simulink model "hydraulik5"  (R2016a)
settings: Solver=ode45  StartTime=0.0  StopTime=2  MaxStep=0.01  RelTol=1e-3  AbsTol=1e-3
InitFcn:
  | pa = 1e5;
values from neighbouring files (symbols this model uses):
  A = zeros(1,N)    [sfun_inferenz.m]
  alpha = 2e-6    (= 2e-06)    [init_epidemie.m]
  m = 1.0    (= 1)    [init_pendelStange.m]
undefined symbols (not defined in the file or in its folder): Amin, K, p0, Qzu, R, rho, ta, te, V0
libraries: simulink x1

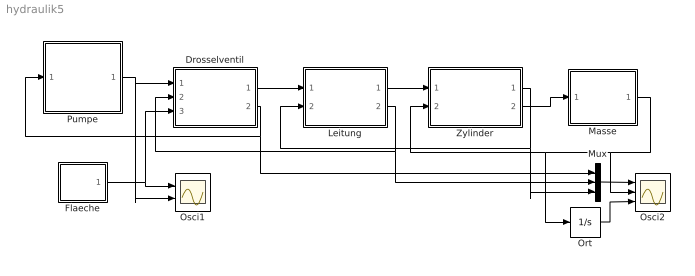
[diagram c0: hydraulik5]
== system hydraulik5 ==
  Drosselventil : Subsystem
  Flaeche : Subsystem
  Leitung : Subsystem
  Masse : Subsystem
  Mux : Mux  Inputs=3
  Ort : Integrator
  Osci1 : Scope  NumInputPorts=2
  Osci2 : Scope  NumInputPorts=3
  Pumpe : Subsystem
  Zylinder : Subsystem
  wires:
  Leitung/2(p1) -> Drosselventil/2(p2), Mux/2
  Leitung/1(Q2) -> Zylinder/1(Q)
  Zylinder/1(p) -> Mux/3, Leitung/2(p2)
  Zylinder/2(F) -> Masse/1(F)
  Masse/1(v) -> Ort/1, Zylinder/2(v), Osci2/2
  Pumpe/1(Q) -> Drosselventil/1(Q1), Osci1/2
  Drosselventil/1(Q2) -> Leitung/1(Q1)
  Drosselventil/2(p1) -> Mux/1, Pumpe/1(p)
  Flaeche/1(Out1) -> Drosselventil/3(A), Osci1/1
  Mux/1 -> Osci2/1
  Ort/1 -> Osci2/3

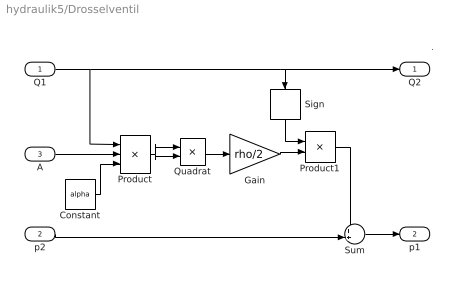
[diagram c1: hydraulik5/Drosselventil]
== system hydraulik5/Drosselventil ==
  note: .
  Q1 : Inport
  p2 : Inport  Port=2
  A : Inport  Port=3
  Constant : Constant  Value=alpha
  Gain : Gain  Gain=rho/2
  Product : Product  Inputs=*//
  Product1 : Product
  Quadrat : Product
  Sign : Signum
  Sum : Sum  Inputs=++|
  Q2 : Outport
  p1 : Outport  Port=2
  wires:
  Sum/1 -> p1/1
  p2/1 -> Sum/2
  Q1/1 -> Product/1, Q2/1, Sign/1
  A/1 -> Product/2
  Constant/1 -> Product/3
  Quadrat/1 -> Gain/1
  Gain/1 -> Product1/2
  Product1/1 -> Sum/1
  Sign/1 -> Product1/1
  Product/1 -> Quadrat/1, Quadrat/2

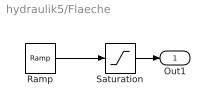
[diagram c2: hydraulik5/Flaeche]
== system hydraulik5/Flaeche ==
  Ramp : simulink/Sources/Ramp  slope=(A-Amin)/(te-ta)  start=ta  X0=0
  Saturation : Saturate  UpperLimit=A  LowerLimit=Amin
  Out1 : Outport
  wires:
  Ramp/1 -> Saturation/1
  Saturation/1 -> Out1/1

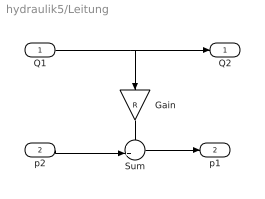
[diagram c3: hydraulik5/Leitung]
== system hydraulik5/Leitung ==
  Q1 : Inport
  p2 : Inport  Port=2
  Gain : Gain  Gain=R
  Sum : Sum  Inputs=++|
  Q2 : Outport
  p1 : Outport  Port=2
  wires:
  Q1/1 -> Q2/1, Gain/1
  p2/1 -> Sum/2
  Sum/1 -> p1/1
  Gain/1 -> Sum/1

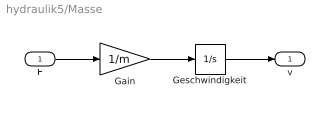
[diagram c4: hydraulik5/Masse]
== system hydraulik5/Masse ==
  F : Inport
  Gain : Gain  Gain=1/m
  Geschwindigkeit : Integrator
  v : Outport
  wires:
  F/1 -> Gain/1
  Geschwindigkeit/1 -> v/1
  Gain/1 -> Geschwindigkeit/1

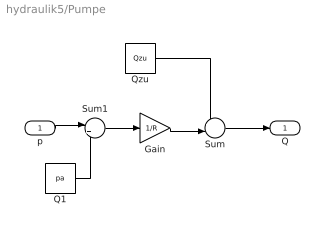
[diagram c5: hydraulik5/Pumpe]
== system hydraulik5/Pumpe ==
  p : Inport
  Gain : Gain  Gain=1/R
  Q1 : Constant  Value=pa
  Qzu : Constant  Value=Qzu
  Sum : Sum  Inputs=+-|
  Sum1 : Sum  Inputs=|+-
  Q : Outport
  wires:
  Qzu/1 -> Sum/1
  Gain/1 -> Sum/2
  Sum/1 -> Q/1
  p/1 -> Sum1/1
  Sum1/1 -> Gain/1
  Q1/1 -> Sum1/2

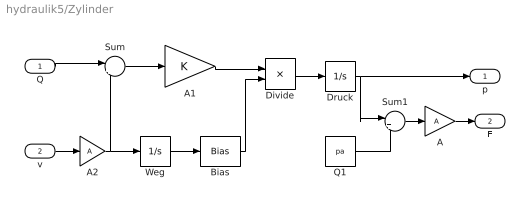
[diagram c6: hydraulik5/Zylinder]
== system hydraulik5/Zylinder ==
  Q : Inport
  v : Inport  Port=2
  A : Gain  Gain=A
  A1 : Gain  Gain=K
  A2 : Gain  Gain=A
  Bias : Bias  Bias=V0
  Divide : Product  Inputs=*/
  Druck : Integrator  InitialCondition=p0  LimitOutput=on  LowerSaturationLimit=0
  Q1 : Constant  Value=pa
  Sum : Sum  Inputs=|+-
  Sum1 : Sum  Inputs=|+-
  Weg : Integrator
  p : Outport
  F : Outport  Port=2
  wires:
  A/1 -> F/1
  Druck/1 -> p/1, Sum1/1
  v/1 -> A2/1
  Weg/1 -> Bias/1
  A2/1 -> Weg/1, Sum/2
  Q/1 -> Sum/1
  Sum/1 -> A1/1
  A1/1 -> Divide/1
  Bias/1 -> Divide/2
  Divide/1 -> Druck/1
  Sum1/1 -> A/1
  Q1/1 -> Sum1/2
